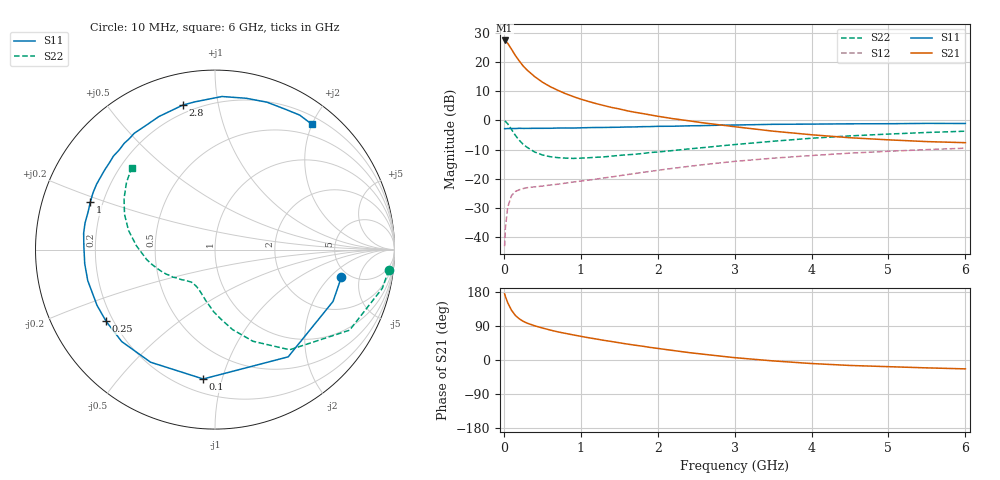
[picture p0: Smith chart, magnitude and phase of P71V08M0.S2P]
! SIEMENS Small Signal Semiconductors
! BFP196
! Si NPN RF Bipolar Junction Transistor in SOT143
! VCE = 1 V  IC = 8 mA
! Common Emitter S-Parameters:  May  1996
# GHz  S  MA  R  50
!  f  S11  S21  S12  S22
! GHz  MAG  ANG  MAG  ANG  MAG  ANG  MAG  ANG
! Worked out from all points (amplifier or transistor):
!   36 points, 10 MHz to 6 GHz, reference 50 ohm
!   highest |S21| = 27.3 dB at 10 MHz (marker M1)
!   |S21| within 3 dB of that: start of sweep to 99.76 MHz
!   unconditionally stable (mu >= 1): 914 MHz to 5.41 GHz; 5.6 GHz to end of sweep
!   at 250 MHz: K = 0.35, MSG = 21.0 dB, |S12| = -23.4 dB
!   at 1.4 GHz: K = 1.17, MAG = 9.4 dB, |S12| = -19.4 dB
!   at 6 GHz: K = 1.01, MAG = 0.2 dB, |S12| = -9.5 dB
!   S11 on the Smith chart (normalised r, x): 10 MHz: 4.31, -2.77; 100 MHz: 0.29, -0.87; 250 MHz: 0.17, -0.29; 1 GHz: 0.15, +0.18; 2.8 GHz: 0.16, +0.79; 6 GHz: 0.32, +2.00
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0.01  0.7207 -12.4  23.3 174.7  0.007 84.8  0.9751 -6.7
0.02  0.7183 -23.7  22.7 167.6  0.0142 80.1  0.957 -13.0
0.05  0.7234 -55.7  20.86 151.3  0.0325 63.9  0.8739 -30.9
0.1  0.7238 -95.2  16.47 131.1  0.0514 47.6  0.6962 -53.3
0.15  0.7229 -119.8  12.87 117.5  0.0604 37.9  0.5528 -67.5
0.2  0.7298 -135.4  10.42 108.8  0.0647 32.6  0.4564 -77.6
0.25  0.7265 -146.6  8.551 102.3  0.0677 29.4  0.389 -85.1
0.3  0.727 -154.7  7.294 97.5  0.0702 28.0  0.3463 -91.2
0.4  0.7297 -166.3  5.611 90.3  0.0726 27.1  0.2872 -100.5
0.5  0.7301 -173.8  4.512 84.5  0.0748 26.9  0.2554 -107.3
0.6  0.7307 178.8  3.786 79.2  0.0779 28.2  0.2386 -112.3
0.7  0.7375 172.9  3.271 74.3  0.0805 29.1  0.2297 -116.9
0.8  0.7391 168.5  2.867 70.3  0.084 30.5  0.2253 -120.9
1  0.7433 159.1  2.304 62.5  0.0911 33.2  0.2249 -126.6
1.1  0.7497 155.1  2.105 58.8  0.0946 34.1  0.2286 -129.0
1.6  0.7691 137.4  1.458 42.2  0.1175 37.8  0.257 -140.6
2.2  0.7917 118.9  1.067 25.1  0.1509 37.6  0.3041 -153.3
2.8  0.8248 102.6  0.838 10.6  0.186 33.9  0.3631 -167.2
3.5  0.8538 87.4  0.652 -2.4  0.2247 26.8  0.4379 177.3
4.5  0.8709 70.5  0.503 -14.4  0.274 16.0  0.5411 158.7
5.5  0.8856 57.8  0.432 -20.8  0.3151 4.7  0.619 142.8
6  0.8826 52.3  0.414 -23.4  0.3332 -1.5  0.651 135.5
